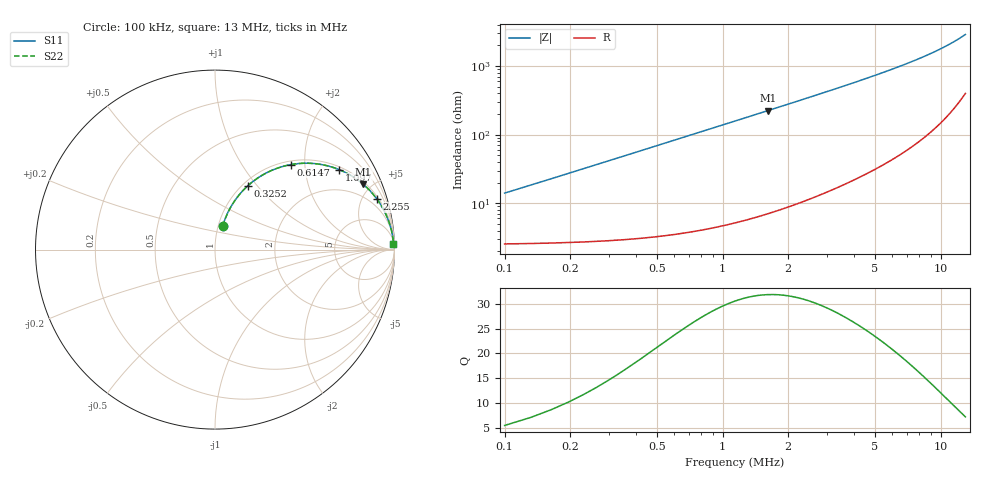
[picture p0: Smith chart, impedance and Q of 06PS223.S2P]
! Coilcraft 0603PS-223 Power Chip Inductor
! 19 February 2003
# MHZ S MA R 50
!Freq  MagS11  AngS11  MagS21  AngS21  MagS12  AngS12  MagS22  AngS22
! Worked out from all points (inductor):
!   402 points, 100 kHz to 13 MHz, reference 50 ohm
!   read as one part in series: L = 22 uH near 164.3 kHz
!   highest Q = 31.9 at 1.612 MHz (marker M1), where L = 22.1 uH
!   S11 on the Smith chart (normalised r, x): 100 kHz: 1.05, +0.28; 325.2 kHz: 1.06, +0.90; 614.7 kHz: 1.07, +1.70; 1.097 MHz: 1.10, +3.04; 2.255 MHz: 1.20, +6.31; 13 MHz: 9, +57
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0.1  0.1358 71.9  0.9664 -7.7  0.9664 -7.7  0.1358 71.9
0.13217  0.1771 71.8  0.9597 -10.1  0.9597 -10.1  0.1771 71.8
0.19651  0.257 69.6  0.9416 -14.8  0.9416 -14.8  0.257 69.6
0.22868  0.2952 68.0  0.9304 -17.1  0.9304 -17.1  0.2952 68.0
0.26085  0.3321 66.3  0.9181 -19.3  0.9181 -19.3  0.3321 66.3
0.32519  0.4012 62.7  0.8906 -23.6  0.8906 -23.6  0.4012 62.7
0.38953  0.464 59.2  0.8603 -27.6  0.8603 -27.6  0.464 59.2
0.45387  0.5204 55.8  0.8282 -31.3  0.8282 -31.3  0.5204 55.8
0.61472  0.6352 48.2  0.7464 -39.4  0.7464 -39.4  0.6352 48.2
0.83991  0.7453 39.8  0.6406 -48.1  0.6406 -48.1  0.7453 39.8
1.09727  0.8233 32.7  0.5412 -55.4  0.5412 -55.4  0.8233 32.7
1.32246  0.8667 28.2  0.4721 -60.0  0.4721 -60.0  0.8667 28.2
1.61199  0.9028 23.7  0.4027 -64.5  0.4027 -64.5  0.9028 23.7
1.90152  0.9261 20.4  0.3494 -67.8  0.3494 -67.8  0.9261 20.4
2.25539  0.9446 17.4  0.2995 -70.7  0.2995 -70.7  0.9446 17.4
3.22049  0.9697 12.3  0.2127 -75.7  0.2127 -75.7  0.9697 12.3
4.41078  0.982 8.8  0.154 -78.9  0.154 -78.9  0.982 8.8
5.40805  0.9869 7.1  0.1233 -80.4  0.1233 -80.4  0.9869 7.1
6.56617  0.9901 5.6  0.09842 -81.4  0.09842 -81.4  0.9901 5.6
8.72156  0.993 3.9  0.06818 -82.2  0.06818 -82.2  0.993 3.9
10.87695  0.9942 2.8  0.04846 -81.8  0.04846 -81.8  0.9942 2.8
13  0.9947 1.9  0.03434 -80.1  0.03434 -80.1  0.9947 1.9
